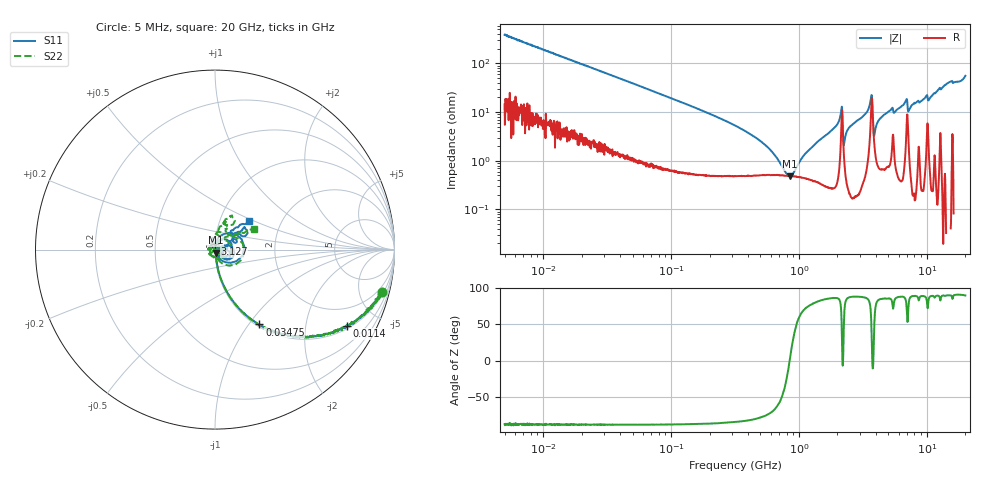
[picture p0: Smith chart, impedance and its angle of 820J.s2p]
!Keysight Technologies,P5008B,MY61100088,A.16.20.02
!Date: Wednesday, November 08, 2023 15:04:16
!Correction: S11(C  2-Port  )
!S21(C  2-Port  )
!S12(C  2-Port  )
!S22(C  2-Port  )
!S2P File: Measurements: S11, S21, S12, S22:Log Frequency Sweep
# Hz S  dB  R 50
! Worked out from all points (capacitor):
!   1601 points, 5 MHz to 20 GHz, reference 50 ohm
!   read as one part in series: C = 82.6 pF near 5.212 MHz
!   lowest |Z| = 484 mohm at 851.1 MHz (marker M1)
!   series resonance near 846 MHz, so ESL is about 430 pH
!   S11 on the Smith chart (normalised r, x): 5 MHz: 1.29, -7.73; 11.4 MHz: 1.11, -3.40; 34.75 MHz: 1.03, -1.13; 3.127 GHz: 1.00, +0.06; 20 GHz: 1.38, +0.47
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5000000  -0.36 -14.4  -12.11 73.5  -12.11 73.5  -0.36 -14.3
1.140052e7  -1.41 -29.9  -6.03 58.1  -6.04 58.1  -1.41 -30.0
1.995555e7  -3.23 -45.0  -3.02 43.6  -3.02 43.6  -3.23 -45.0
3.474974e7  -6.29 -59.3  -1.31 28.9  -1.31 28.9  -6.29 -59.4
7.964482e7  -12.48 -74.7  -0.31 13.6  -0.31 13.6  -12.50 -74.9
3.162278e8  -24.60 -81.9  -0.06 2.7  -0.06 2.7  -24.95 -83.3
8.5113e8  -34.66 -73.4  -0.05 -0.9  -0.05 -0.9  -39.42 -82.5
1.149663e9  -39.60 -66.3  -0.06 -1.9  -0.06 -1.9  -60.24 -128.8
1.2621e9  -41.18 -66.0  -0.06 -2.3  -0.06 -2.3  -55.83 142.1
1.593682e9  -56.25 19.7  -0.06 -3.4  -0.06 -3.4  -40.53 106.6
2.119447e9  -25.50 67.9  -0.24 -7.0  -0.24 -7.0  -25.37 65.0
2.387823e9  -51.80 120.3  -0.07 -4.7  -0.08 -4.7  -46.57 141.7
3.126577e9  -30.25 92.7  -0.07 -7.6  -0.07 -7.6  -33.04 76.1
3.690713e9  -15.95 21.2  -1.39 -11.7  -1.39 -11.7  -16.05 12.7
4.334113e9  -49.02 -26.3  -0.06 -8.8  -0.06 -8.8  -39.24 -45.0
5.037181e9  -38.21 51.2  -0.06 -11.2  -0.06 -11.2  -35.47 36.6
5.332756e9  -32.22 46.5  -0.14 -12.5  -0.14 -12.5  -30.33 28.8
5.793917e9  -37.80 -20.1  -0.05 -12.7  -0.05 -12.7  -47.60 82.8
7.018914e9  -19.17 -9.7  -0.78 -16.1  -0.78 -16.1  -25.21 -19.9
9.629383e9  -28.76 -19.9  -0.02 -22.8  -0.02 -22.8  -33.43 164.7
1.457812e10  -14.12 36.6  -0.09 -36.3  -0.09 -36.3  -14.34 67.6
2e10  -12.13 39.9  -0.31 -56.6  -0.31 -56.5  -12.26 27.7
